|//////////////////////////////////////////////////////////////////////////////
|//////////////////////////////////////////////////////////////////////////////
|   @@@@@@@   @@@@@@@   @@@@@@@   @@@@@@@   @@@@@@@   @@@@@@   @@
|   @@@@@@@@@   @@@@@@@@@   @@@@@@@@@   @@@@@@@@@   @@@@@@@@@ @@@@@@@@  @
|   @@@   @@@ @@@   @@@ @@@   @@@   @@@ @@@   @@@@   @@@  @
|   @@   @@ @@   @@ @@@@@@@@@@@ @@@@@@@@@@@ @@   @@   @@ @@
|   @@@   @@@ @@   @@   @@@ @@@   @@   @@   @@ @@
|   @@@@@@@@@  @@   @@  @@@@@@@@@   @@@@@@@@@  @@   @@   @@ @@
|   @@@@@@@   @@   @@   @@@@@@@   @@@@@@@   @@   @@   @@ @@
|   IBIS Model of NL3V8T244
|   8-Bit Dual-Supply Level Translator
|   Package Type: UDFN20, CASE 517AK
|   TSSOP-20 WB, CASE 948E
|   SOIC-20 WB, CASE 751D-05
|   The model is covering the following Vccs:
|   0.9V, 1.2V, 1.5V, 1.8V, 2.5V, 3.3V
|//////////////////////////////////////////////////////////////////////////////
|//////////////////////////////////////////////////////////////////////////////
[IBIS Ver]   3.2
|   7.2 compatible
|//////////////////////////////////////////////////////////////////////////////
[Comment Char] |_char
|//////////////////////////////////////////////////////////////////////////////
[File Name]   nl3v8t244_va_r0.ibs
|//////////////////////////////////////////////////////////////////////////////
[File Rev]   0.0
|   0.0 - May 23, 2025 - File created
|//////////////////////////////////////////////////////////////////////////////
[Date]   May 23, 2025
|//////////////////////////////////////////////////////////////////////////////
[Source]   From lab measurements and simulations at onsemi
|//////////////////////////////////////////////////////////////////////////////
[Notes]   - The currents greater than +/- 100 mA are extrapolated
|//////////////////////////////////////////////////////////////////////////////
[Disclaimer]
   - onsemi Corporation hereby grants
   the user of this IBIS model a license to use this model
   under the following terms. This license is nonexclusive
   and nontransferable. Before using this IBIS model.
   After reading the terms and conditions of this license,
   the user either must accept these terms,
   or the IBIS model should be returned to onsemi within 30 days.
   - The user is hereby granted a license to use the IBIS model.
   This shall not be construed as a right to sell,
   or otherwise profit either by leasing or renting this software.
   - The user may modify the IBIS model to suit his specific
   applications but rights to derivative works and such
   modifications shall belong to onsemi.
   - This IBIS model is provided on an "as is" basis.
   onsemi makes absolutely no warranty with respect
   to the information contained herein.
   By use of this IBIS model, the user assumes full risk as to the
   quality and suitablility of the model to his particular use,
   and by using this model assumes the entire risk.
   Under all circumstances the user shall not hold
   onsemi liable in any way for the results obtained.
   onsemi reserves the right to make to improve
   the model for reliability, function, or design.
   onsemi does not convey any license under patent
   rights or any other intellectual property rights,
   including those of third parties.
   - onsemi is not obligated to provide maintenance
   or support for the licensed IBIS model.
   - Cont onsemi at ATTN:LOGIC APPLICATIONS/IBIS MODEL.
   5701 N Pima Rd, Scottsdale, AZ 85250
|//////////////////////////////////////////////////////////////////////////////
[Copyright]   (c) 2025 onsemi Corp.
|//////////////////////////////////////////////////////////////////////////////
|//////////////////////////////////////////////////////////////////////////////
[Component]   NL3V8T244DWR2G
|//////////////////////////////////////////////////////////////////////////////
[Manufacturer]  onsemi
|   Data Sheet: NL3V8T244/D, March, 2024 - Rev. P0
|//////////////////////////////////////////////////////////////////////////////
[Package]
|   SOIC-20 WB
| CASE 751D-05
|  DW SUFFIX
|variable   typ   min   max
R_pkg   0.0388   0.0342   0.0456
L_pkg   5.0121nH   4.1117nH   6.34108nH
C_pkg   0.7179pF   0.532pF   0.8692pF
[Pin] signal_name   model_name   R_pin   L_pin   C_pin
1   VCCA   POWER   0.0438   6.3361nH   0.8661pF
2   A1   In1   0.0438   5.5422nH   0.8677pF
3   A2   In1   0.0352   4.7156nH   0.7335pF
4   A3   In1   0.0358   4.3786nH   0.5920pF
5   A4   In1   0.0362   4.1319nH   0.5345pF
6   A5   In1   0.0352   4.1126nH   0.5320pF
7   A6   In1   0.0346   4.2858nH   0.5830pF
8   A7   In1   0.0343   4.6345nH   0.7277pF
9   A8   In1   0.0450   5.5191nH   0.8670pF
10   GND   GND   0.0431   6.3411nH   0.8676pF
11   OE   In2   0.0426   6.2822nH   0.8618pF
12   B8   Out   0.0456   5.5625nH   0.8610pF
13   B7   Out   0.0347   4.7792nH   0.7424pF
14   B6   Out   0.0364   4.4145nH   0.5967pF
15   B5   Out   0.0353   4.1117nH   0.5339pF
16   B4   Out   0.0378   4.1320nH   0.5337pF
17   B3   Out   0.0343   4.3776nH   0.5922pF
18   B2   Out   0.0342   4.7153nH   0.7314pF
19   B1   Out   0.0442   5.5610nH   0.8692pF
20   VCCB   POWER   0.0438   6.3083nH   0.8641pF
|//////////////////////////////////////////////////////////////////////////////
|//////////////////////////////////////////////////////////////////////////////
[Component]   NL3V8T244DTR2G
|//////////////////////////////////////////////////////////////////////////////
[Manufacturer]  onsemi
|   Data Sheet: NL3V8T244/D, March, 2024 - Rev. P0
|//////////////////////////////////////////////////////////////////////////////
[Package]
|   TSSOP-20 WB
| CASE 948E
|  DT SUFFIX
| variable   typ   min   max
R_pkg   0.0419   0.0344   0.0490
L_pkg   0.4237nH   0.3470nH   0.5107nH
C_pkg   0.1104pF   0.1061pF   0.1153pF
|//////////////////////////////////////////////////////////////////////////////
[Pin] signal_name   model_name   R_pin   L_pin   C_pin
1   VCCA   POWER   0.0421   0.4133nH   0.1099pF
2   A1   In1   0.0344   0.3470nH   0.1061pF
3   A2   In1   0.0443   0.4580nH   0.1121pF
4   A3   In1   0.0490   0.5107nH   0.1153pF
5   A4   In1   0.0004   0.0379nH   0.0765pF
6   A5   In1   0.0438   0.4489nH   0.1118pF
7   A6   In1   0.0421   0.4133nH   0.1099pF
8   A7   In1   0.0344   0.3470nH   0.1061pF
9   A8   In1   0.0443   0.4580nH   0.1121pF
10   GND   GND   0.0490   0.5107nH   0.1153pF
11   OE   In2   0.0004   0.0379nH   0.0765pF
12   B8   Out   0.0438   0.4489nH   0.1118pF
13   B7   Out   0.0421   0.4133nH   0.1099pF
14   B6   Out   0.0344   0.3470nH   0.1061pF
15   B5   Out   0.0443   0.4580nH   0.1121pF
16   B4   Out   0.0490   0.5107nH   0.1153pF
17   B3   Out   0.0004   0.0379nH   0.0765pF
18   B2   Out   0.0438   0.4489nH   0.1118pF
19   B1   Out   0.0004   0.0379nH   0.0765pF
20   VCCB   POWER   0.0438   0.4489nH   0.1118pF
|//////////////////////////////////////////////////////////////////////////////
|//////////////////////////////////////////////////////////////////////////////
[Component]   NL3V8T244MU2TAG
|//////////////////////////////////////////////////////////////////////////////
[Manufacturer]  onsemi
|   Data Sheet: NL3V8T244/D, March, 2024 - Rev. P0
|//////////////////////////////////////////////////////////////////////////////
[Package]
|   UDFN20
| CASE 517AK
|  MU SUFFIX
| variable   typ   min   max
R_pkg   0.0510   0.0410   0.0590
L_pkg   1.1228nH   1.0268nH   1.27nH
C_pkg   0.3524pF   0.34108pF   0.364pF
|//////////////////////////////////////////////////////////////////////////////
[Pin] signal_name   model_name   R_pin   L_pin   C_pin
1   VCCA   POWER   0.0526   1.1676nH   0.3611pF
2   A1   In1   0.0477   1.0491nH   0.3458pF
3   A2   In1   0.0490   1.0555nH   0.3452pF
4   A3   In1   0.0512   1.1110nH   0.3515pF
5   A4   In1   0.0565   1.2271nH   0.3610pF
6   A5   In1   0.0532   1.1681nH   0.3565pF
7   A6   In1   0.0410   1.0883nH   0.3495pF
8   A7   In1   0.0483   1.0553nH   0.3461pF
9   A8   In1   0.0411   1.0915nH   0.3498pF
10   GND   GND   0.0549   1.1846nH   0.3637pF
11   OE   In2   0.0547   1.1827nH   0.3620pF
12   B8   Out   0.0550   1.1086nH   0.3411pF
13   B7   Out   0.0496   1.0770nH   0.3490pF
14   B6   Out   0.0590   1.1079nH   0.3497pF
15   B5   Out   0.0549   1.2700nH   0.3631pF
16   B4   Out   0.0512   1.1423nH   0.3571pF
17   B3   Out   0.0480   1.0438nH   0.3456pF
18   B2   Out   0.0476   1.0268nH   0.3460pF
19   B1   Out   0.0496   1.0940nH   0.3411pF
20   VCCB   POWER   0.0559   1.2042nH   0.3640pF
|//////////////////////////////////////////////////////////////////////////////
|//////////////////////////////////////////////////////////////////////////////
[Model Selector]   In1
In1_09   Vcc = 0.90
In1_12   Vcc = 1.20
In1_15   Vcc = 1.50
In1_18   Vcc = 1.80
In1_25   Vcc = 2.50
In1_33   Vcc = 3.30
|//////////////////////////////////////////////////////////////////////////////
[Model Selector]   In2
In2_09   Vcc = 0.90
In2_12   Vcc = 1.20
In2_15   Vcc = 1.50
In2_18   Vcc = 1.80
In2_25   Vcc = 2.50
In2_33   Vcc = 3.30
|//////////////////////////////////////////////////////////////////////////////
[Model Selector]   Out
Out_09   Vcc = 0.90
Out_12   Vcc = 1.20
Out_15   Vcc = 1.50
Out_18   Vcc = 1.80
Out_25   Vcc = 2.50
Out_33   Vcc = 3.30
| Models and submodels in the file (18): In1_09 (Input), In2_09 (Input), Out_09 (3-state), In1_12 (Input), In2_12 (Input), Out_12 (3-state), In1_15 (Input), In2_15 (Input), Out_15 (3-state), In1_18 (Input), In2_18 (Input), Out_18 (3-state), In1_25 (Input), In2_25 (Input), Out_25 (3-state), In1_33 (Input), In2_33 (Input), Out_33 (3-state)
